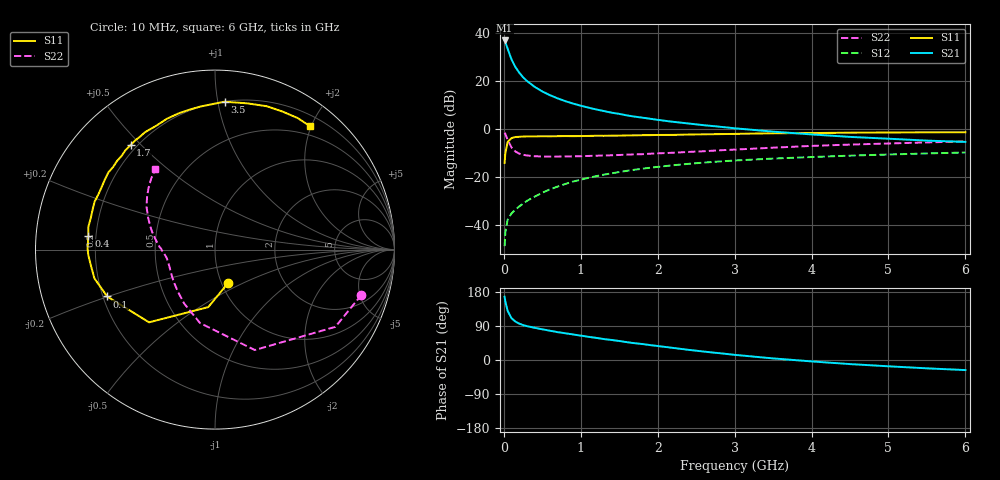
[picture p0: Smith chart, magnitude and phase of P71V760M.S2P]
! SIEMENS Small Signal Semiconductors
! BFP196
! Si NPN RF Bipolar Junction Transistor in SOT143
! VCE = 1.75 V  IC = 60 mA
! Common Emitter S-Parameters:  May  1996
# GHz  S  MA  R  50
!  f  S11  S21  S12  S22
! GHz  MAG  ANG  MAG  ANG  MAG  ANG  MAG  ANG
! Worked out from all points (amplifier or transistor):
!   36 points, 10 MHz to 6 GHz, reference 50 ohm
!   highest |S21| = 37.0 dB at 10 MHz (marker M1)
!   |S21| within 3 dB of that: start of sweep to 44.48 MHz
!   unconditionally stable (mu >= 1): 363.7 MHz to 4.623 GHz
!   at 250 MHz: K = 0.90, MSG = 26.3 dB, |S12| = -30.9 dB
!   at 1.4 GHz: K = 1.10, MAG = 10.7 dB, |S12| = -18.3 dB
!   at 6 GHz: K = 0.99, MSG = 2.2 dB, |S12| = -9.7 dB
!   S11 on the Smith chart (normalised r, x): 10 MHz: 1.07, -0.42; 100 MHz: 0.22, -0.20; 400 MHz: 0.17, +0.05; 1.7 GHz: 0.18, +0.47; 3.5 GHz: 0.20, +1.05; 6 GHz: 0.36, +1.98
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0.01  0.2 -68.6  70.4 166.9  0.0037 78.6  0.8541 -17.2
0.02  0.3227 -96.7  64.88 154.0  0.0073 67.8  0.7967 -32.7
0.05  0.5469 -132.2  46.96 129.2  0.0132 54.2  0.6018 -68.4
0.1  0.6551 -156.5  28.31 110.3  0.0178 49.5  0.4176 -101.5
0.15  0.6908 -166.6  19.73 101.4  0.0214 51.3  0.3454 -120.0
0.2  0.697 -172.6  15.05 96.0  0.0248 54.4  0.3116 -131.8
0.25  0.7065 -177.5  12.07 92.2  0.0284 57.0  0.294 -140.3
0.3  0.71 179.6  10.11 89.4  0.0324 59.4  0.2851 -146.0
0.4  0.7098 173.8  7.647 84.9  0.0396 62.2  0.2751 -154.3
0.5  0.7171 169.9  6.118 81.0  0.0479 63.7  0.271 -159.5
0.6  0.7142 165.7  5.11 77.2  0.0563 64.2  0.2703 -163.0
0.7  0.718 161.3  4.392 73.5  0.0643 64.3  0.2709 -165.9
0.9  0.7188 154.5  3.425 67.4  0.0818 62.6  0.2729 -170.0
1.1  0.7267 147.8  2.817 61.2  0.0977 61.2  0.2788 -173.0
1.3  0.7308 140.9  2.393 55.3  0.1138 58.4  0.2844 -175.7
1.7  0.7484 128.9  1.834 44.3  0.144 52.8  0.2999 179.1
2.2  0.7637 115.4  1.429 31.9  0.1785 45.1  0.3251 173.0
2.8  0.7925 100.3  1.133 18.0  0.2138 36.0  0.3647 164.1
3.5  0.8256 86.3  0.893 4.2  0.2458 26.0  0.4141 154.3
4.5  0.8494 70.1  0.694 -10.8  0.2827 13.9  0.4801 142.0
5.5  0.8656 57.9  0.581 -22.0  0.3143 3.1  0.5332 131.7
6  0.8676 52.5  0.546 -26.6  0.3287 -2.7  0.558 126.6
